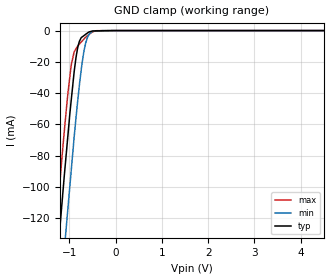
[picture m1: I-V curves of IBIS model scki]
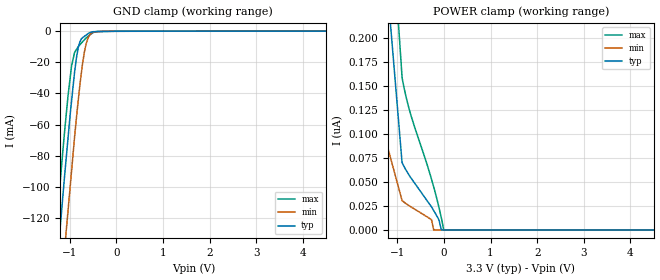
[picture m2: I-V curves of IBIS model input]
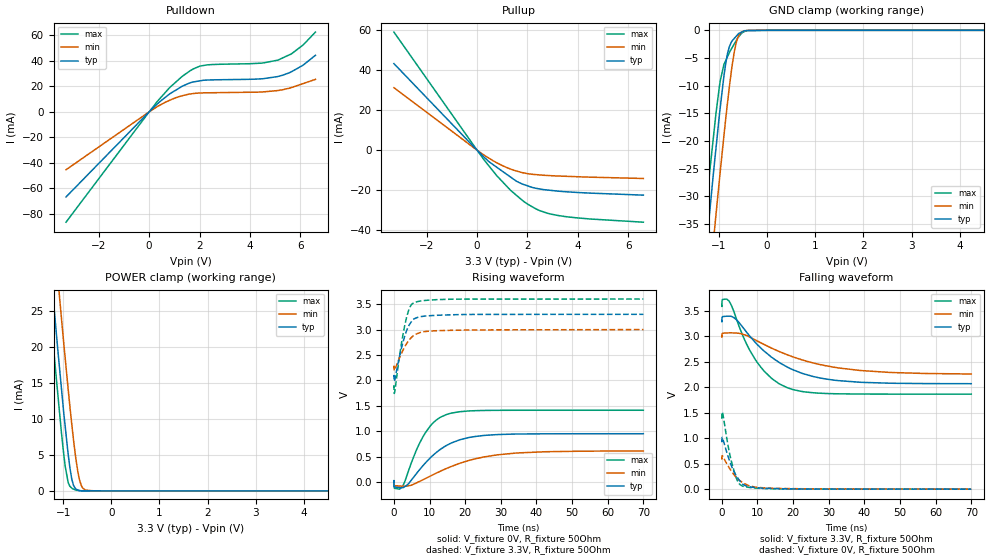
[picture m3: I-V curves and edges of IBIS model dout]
|Texas Instruments Incorporated
| 99dB SNR Stereo ADC with Single-Ended Inputs
| Marketing part#   Digital Voltage Range   Package-type   #pins
| PCM1808PW   2.7V-3.6V   TSSOP   14
| PCM1808PWG4   2.7V-3.6V   TSSOP   14
| PCM1808PWR   2.7V-3.6V   TSSOP   14
| PCM1808PWRG4   2.7V-3.6V   TSSOP   14
[IBIS Ver]   3.2
[File name]   pcm1808.ibs
[File Rev]   1.0
[Date]   1/17/2012
[Source]
| Texas Instruments Incorporated.
| Analog-eLab Design Center, HPA
| 12500 TI Blvd
| Dallas, TX -75243
| e-mail: elab_scm_ibis@list.ti.com
[Notes]   Revision History:
| Rev 1.0: 1/17/2012
| - Initial version of the model
| - Model generated from simulations in HSPICE
| - Model matched to SPICE simulation
| - C_comp although listed in numerical order of value are
|   obtained from varying PVT conditions. For PVT conditions for
|   each specific value refer the buffer description under
|   respective [Model]. IBIS model user is responsible for using
|   appropriate C_comp to simulate for Signal Integrity.
|*  EXCEPTION:   *
|*  - For model scki and io, there will be a leakage current in the GND *
|*   clamp I-V Table.   *
[Disclaimer]
| This model is designed as an aid for customers of Texas Instruments.
| TI and its licensors and suppliers make no warranties, either expressed
| or implied, with respect to this  model, including the warranties of
| merchantability or fitness for a particular purpose. The model is
| provided solely on an "as is" basis. The entire risk as to its quality
| and performance is with the customer.
[Copyright]
 (C) Copyright 2011 Texas Instruments Incorporated.All rights reserved.
|   PCM1808
[Component]   PCM1808
[Manufacturer]   TI
[Package]   |14 TSSOP   -  PW package
|   typ   min   max
R_pkg   0.18553   0.14171   0.22788
L_pkg   2.94018nH   2.37771nH   3.60093nH
C_pkg   0.47240pF   0.43357pF   0.52376pF
[Pin]  signal_name   model_name   R_pin   L_pin   C_pin
1   VREF   term   0.22788   3.60093nH  0.52303pF
2   AGND   gnd   0.20058   2.85057nH  0.45502pF
3   VCC   power   0.15622   2.49388nH  0.43728pF
4   VDD   power   0.14794   2.42818nH  0.43189pF
5   DGND   gnd   0.14149   2.37678nH  0.43593pF
6   SCKI   scki   0.15718   2.50766nH  0.43740pF
7   LRCK   io   0.19988   3.36685nH  0.51135pF
8   BCK   io   0.19821   3.35423nH  0.51130pF
9   DOUT   dout   0.16646   2.57842nH  0.44041pF
10   MD0   input   0.16820   2.58778nH  0.44682pF
11   MD1   input   0.14171   2.37771nH  0.43357pF
12   FMT   input   0.16963   2.59944nH  0.44279pF
13   VINL   term   0.19942   2.83905nH  0.45353pF
14   VINR   term   0.22675   3.58976nH  0.52376pF
[Model] term
Model_type Terminator
C_comp   1.0e-20F  1.0e-20F  1.0e-20F
|   typ   min   max
[Voltage Range]   3.3V   3.0V   3.6V
[POWER Clamp Reference]   3.3V   3.0V   3.6V
[GND Clamp Reference]   0V   0V   0V
|Ambient Temperature   25   85   -40
|Junction Temperature
[Temperature Range]   27   125   -40
| Models and submodels in the file (5): scki (Input), input (Input), dout (3-state), io (I/O), term (Terminator)
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|   scki Model
[Model]   scki
Model_type   Input
Vinl = 0.8
Vinh = 2.0
|   typ   min   max
|   (nom PVT)   (fast PVT)   (slow PVT)
C_comp   1.546e-12   1.133e-12   1.608e-12
| Where nom  PVT is Nominal Process, 3.3V, 27C
|   Fast PVT is Strong Process,  3.6V, -40C
|   Slow PVT is Weak Process,   3V, 125C
[Voltage Range]   3.3   3   3.6
|Ambient Temperature   25   85   -40
|Junction Temperature
[Temperature Range]   27   125   -40
[Power Clamp Reference]   3.3   3   3.6
[GND Clamp Reference]   0   0   0
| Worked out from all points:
|   GND clamp passes 1 mA (typ) near -0.58 V on its own axis
[GND Clamp]
|   Voltage   I(typ)   I(min)   I(max)
-3.3V     -909.9mA   -953.5mA   -882.6mA
-1.336V   -172.6mA   -220.3mA   -142.8mA
-1.284V   -153.7mA   -201.5mA   -124.5mA
-1.159V   -109.9mA   -156.6mA   -80.59mA
-1.109V   -92.22mA   -139.5mA   -63.74mA
-1.04V    -69.7mA    -116.4mA   -42.33mA
-961.2mV  -44.7mA    -89.67mA   -22.09mA
-858mV    -17.33mA   -55.94mA   -11.7mA
-732mV    -4.257mA   -22.14mA   -6.932mA
-590.7mV  -1.106mA   -3.229mA   -2.814mA
-285mV    -137.9uA   -2.979uA   -46.26uA
6.6V      0A         0A         0A
[POWER Clamp]
|   Voltage   I(typ)   I(min)   I(max)
-3.3V     0A         0A         0A
6.6V      0A         0A         0A
|   input Model
[Model]   input
Model_type   Input
Vinl = 0.8
Vinh = 2.0
|   typ   min   max
|   (nom PVT)   (fast PVT)   (slow PVT)
C_comp   1.569e-12   1.148e-12   1.633e-12
| Where nom  PVT is Nominal Process, 3.3V, 27C
|   Fast PVT is Strong Process,  3.6V, -40C
|   Slow PVT is Weak Process,   3V, 125C
[Voltage Range]   3.3   3   3.6
|Ambient Temperature   25   85   -40
|Junction Temperature
[Temperature Range]   27   125   -40
[Power Clamp Reference]   3.3   3   3.6
[GND Clamp Reference]   0   0   0
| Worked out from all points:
|   GND clamp passes 1 mA (typ) near -0.58 V on its own axis
[GND Clamp]
|   Voltage   I(typ)   I(min)   I(max)
-3.3V     -909.9mA   -953.5mA   -882.6mA
-1.336V   -172.6mA   -220.3mA   -142.8mA
-1.284V   -153.7mA   -201.5mA   -124.5mA
-1.159V   -109.9mA   -156.6mA   -80.6mA
-1.109V   -92.22mA   -139.5mA   -63.76mA
-1.04V    -69.71mA   -116.4mA   -42.36mA
-961.2mV  -44.71mA   -89.68mA   -22.13mA
-858mV    -17.35mA   -55.94mA   -11.76mA
-732mV    -4.28mA    -22.15mA   -6.966mA
-590.7mV  -1.132mA   -3.239mA   -2.842mA
-285mV    -152.1uA   -11.23uA   -66.02uA
6.6V      65.17uA    30.87uA    124.2uA
[POWER Clamp]
|   Voltage   I(typ)   I(min)   I(max)
-3.3V     12.17uA    4.486uA    29.58uA
-1.746V   564.6nA    208.6nA    1.42uA
-1.674V   522.7nA    170.8nA    1.161uA
-1.397V   361.2nA    120.8nA    521nA
-897.6mV  70.47nA    30.77nA    159.8nA
-716.4mV  55.03nA    24.42nA    121.3nA
-264mV    23.96nA    10.53nA    52.71nA
-219.6mV  20.28nA    0A         45.12nA
-104.4mV  10.29nA    0A         23.21nA
-54mV     0A         0A         12.48nA
-3.3mV    0A         0A         0A
6.6V      0A         0A         0A
|   dout Model
[Model]   dout
Model_type   3-state
Polarity   Non-Inverting
Vmeas = 1.65
Vref = 1.65
Cref = 20pF
Rref = 50
|   typ   min   max
|   (nom PVT)   (fast PVT)   (slow PVT)
C_comp   1.530e-12   1.486e-12   1.584e-12
|ON state : BUFFER OUTPUT TURNED HIGH
|C_comp   1.530e-12   1.486e-12   1.584e-12
|OFF state: BUFFER IN HIGH IMPEDANCE
|C_comp   1.241e-12   1.198e-12   1.327e-12
| Where nom  PVT is Nominal Process, 3.3V, 27C
|   Fast PVT is Strong Process,  3.6V, -40C
|   Slow PVT is Weak Process,   3V, 125C
[Voltage Range]   3.3   3   3.6
|Ambient Temperature   25   85   -40
|Junction Temperature
[Temperature Range]   27   125   -40
[Pullup Reference]   3.3   3   3.6
[Pulldown Reference]   0   0   0
[Power Clamp Reference]   3.3   3   3.6
[GND Clamp Reference]   0   0   0
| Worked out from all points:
|   slope of the pulldown table from 0 to 0.495 V, typ, clamps not added: 54.1 ohm
|   slope of the pullup table from 0 to 0.495 V, typ, clamps not added: 83.3 ohm
|   GND clamp passes 1 mA (typ) near -0.64 V on its own axis
|   POWER clamp passes 1 mA (typ) near -0.79 V on its own axis
|   falling waveform, V_fixture 3.3V, R_fixture 50Ohm: 20-80 % time 13.7ns typ, 18.8ns min, 8.86ns max; typ from 3.3 V to 2.07 V
|   rising waveform, V_fixture 0V, R_fixture 50Ohm: 20-80 % time 9.29ns typ, 14.6ns min, 6.15ns max; typ from 0 V to 0.951 V
|   rising waveform, V_fixture 3.3V, R_fixture 50Ohm: 20-80 % time 2.94ns typ, 3.66ns min, 2.56ns max; typ from 2.07 V to 3.3 V
|   falling waveform, V_fixture 0V, R_fixture 50Ohm: 20-80 % time 3.52ns typ, 4.53ns min, 2.69ns max; typ from 0.951 V to 0 V
[Pulldown]
|   Voltage   I(typ)   I(min)   I(max)
-3.3V     -66.69mA   -45.36mA   -86.43mA
327.6mV   6.272mA    4.171mA    8.266mA
831.6mV   14.32mA    9.217mA    19.32mA
1.307V    20.02mA    12.6mA     27.74mA
1.709V    23.3mA     14.26mA    33.15mA
2.023V    24.33mA    14.8mA     35.91mA
2.477V    25.04mA    14.99mA    37.06mA
4.471V    25.9mA     15.58mA    38.2mA
5.112V    27.73mA    16.71mA    40.56mA
5.648V    31.46mA    19.05mA    45.47mA
6.116V    36.71mA    22.21mA    52.52mA
6.6V      44.33mA    25.47mA    62.51mA
[GND Clamp]
|   Voltage   I(typ)   I(min)   I(max)
-3.3V     -235.3mA   -247mA     -228mA
-1.364V   -48.58mA   -60.96mA   -40.92mA
-1.287V   -41.34mA   -53.77mA   -33.98mA
-1.195V   -33.04mA   -45.33mA   -25.76mA
-1.112V   -25.52mA   -37.79mA   -19.03mA
-1.062V   -21.27mA   -33.27mA   -14.98mA
-972mV    -13.82mA   -25.36mA   -9.036mA
-821.7mV  -4.161mA   -13.01mA   -4.737mA
-675mV    -1.39mA    -3.55mA    -2.351mA
-600mV    -655.6uA   -1.129mA   -1.279mA
-501mV    -198.3uA   -164.7uA   -351.3uA
6.6V      0A         0A         0A
[Pullup]
|   Voltage   I(typ)   I(min)   I(max)
-3.3V     43.14mA    31.15mA    58.85mA
327.6mV   -4.056mA   -2.874mA   -5.625mA
788.4mV   -8.565mA   -6.315mA   -12.79mA
1.332V    -13.42mA   -9.422mA   -20.02mA
1.558V    -15.43mA   -10.38mA   -22.44mA
1.818V    -16.96mA   -11.25mA   -25.22mA
2.477V    -19.29mA   -12.32mA   -30.06mA
2.822V    -19.89mA   -12.62mA   -31.52mA
3.244V    -20.45mA   -12.88mA   -32.61mA
4.471V    -21.38mA   -13.44mA   -34.27mA
6.6V      -22.4mA    -14.1mA    -35.88mA
[POWER Clamp]
|   Voltage   I(typ)   I(min)   I(max)
-3.3V     193.3mA    202.3mA    187.7mA
-1.29V    33.04mA    43.04mA    26.79mA
-1.17V    23.99mA    33.88mA    17.63mA
-1.112V   19.65mA    29.6mA     13.51mA
-1.04V    14.56mA    24.32mA    8.399mA
-957.6mV  8.946mA    18.4mA     3.427mA
-896.4mV  5.109mA    14.14mA    1.179mA
-818.4mV  1.584mA    9.088mA    378.2uA
-738mV    287.1uA    4.567mA    118.4uA
-627mV    22.65uA    817.6uA    19.77uA
-534mV    19.27uA    109.1uA    4.598uA
6.6V      0A         0A         0A
[Ramp]
R_load = 50
|   typ   min   max
dV/dt_r   0.570804/9.28996e-09   0.367474/1.46039e-08   0.847978/6.15152e-09
dV/dt_f   0.739432/1.36256e-08   0.445442/1.87455e-08   1.04207/8.82963e-09
[Falling Waveform]
V_fixture = 3.3V
V_fixture_min = 3V
V_fixture_max = 3.6V
R_fixture = 50Ohm
|   Time   V(typ)   V(min)   V(max)
0s        3.3V       3V         3.6V
168ps     3.38V      3.054V     3.716V
1.976ns   3.392V     3.064V     3.692V
3.468ns   3.359V     3.063V     3.466V
6.412ns   3.127V     3.025V     2.925V
9.476ns   2.87V      2.923V     2.532V
13.78ns   2.597V     2.772V     2.184V
18.52ns   2.388V     2.63V      1.985V
32.64ns   2.128V     2.378V     1.87V
70ns      2.068V     2.258V     1.863V
[Rising Waveform]
V_fixture = 0V
V_fixture_min = 0V
V_fixture_max = 0V
R_fixture = 50Ohm
|   Time   V(typ)   V(min)   V(max)
0s        0V         0V         0V
164ps     -93.95mV   -66.97mV   -120.7mV
2.144ns   -111.3mV   -79.23mV   -105.3mV
4.212ns   -22.86mV   -71.13mV   246.1mV
8.752ns   370.9mV    67.23mV    961.8mV
11.83ns   579.2mV    174mV      1.217V
14.98ns   729.2mV    274.5mV    1.335V
21.48ns   882.3mV    433.7mV    1.401V
33.8ns    944.7mV    568.6mV    1.413V
70ns      951.3mV    612.5mV    1.413V
[Rising Waveform]
V_fixture = 3.3V
V_fixture_min = 3V
V_fixture_max = 3.6V
R_fixture = 50Ohm
|   Time   V(typ)   V(min)   V(max)
0s        2.067V     2.253V     1.863V
4ps       2.097V     2.281V     1.894V
68ps      1.991V     2.208V     1.751V
216ps     2.004V     2.202V     1.772V
1.976ns   2.594V     2.509V     2.666V
3.564ns   2.978V     2.723V     3.243V
4.516ns   3.115V     2.815V     3.444V
5.932ns   3.22V      2.901V     3.536V
16.03ns   3.291V     2.985V     3.597V
70ns      3.3V       3V         3.6V
[Falling Waveform]
V_fixture = 0V
V_fixture_min = 0V
V_fixture_max = 0V
R_fixture = 50Ohm
|   Time   V(typ)   V(min)   V(max)
0s        951.3mV    613mV      1.413V
68ps      1.007V     646.5mV    1.505V
216ps     1.004V     651.8mV    1.493V
2.14ns    561.9mV    410.7mV    712.3mV
3.564ns   322.5mV    271.7mV    327.4mV
4.516ns   213.4mV    200.1mV    143.4mV
5.932ns   94.69mV    124.6mV    57.44mV
9.18ns    31.85mV    43.28mV    22.82mV
14.44ns   13.03mV    18.36mV    6.989mV
70ns      585.8nV    29.01uV    0V
